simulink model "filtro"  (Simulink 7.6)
settings: Solver=ode45  StartTime=0.0  StopTime=100  MaxStep=0.1  RelTol=1e-3  AbsTol=1e-3

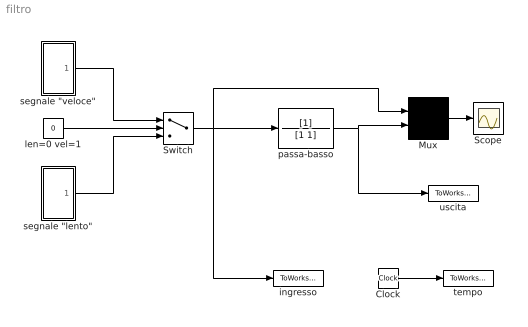
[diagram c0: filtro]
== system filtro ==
  Clock : Clock
  Mux : Mux  Inputs=2
  Scope : Scope
  Switch : Switch  Threshold=1
  ingresso : ToWorkspace  VariableName=u  SaveFormat=Array
  len=0 vel=1 : Constant  Value=0
  passa-basso : TransferFcn  Denominator=[1 1]
  "segnale \"lento\"" : Subsystem
  "segnale \"veloce\"" : Subsystem
  tempo : ToWorkspace  VariableName=t  SaveFormat=Array
  uscita : ToWorkspace  VariableName=yf  SaveFormat=Array
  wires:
  Mux/1 -> Scope/1
  Clock/1 -> tempo/1
  passa-basso/1 -> Mux/2, uscita/1
  len=0 vel=1/1 -> Switch/2
  "segnale \"veloce\""/1(out_1) -> Switch/1
  "segnale \"lento\""/1(out_1) -> Switch/3
  Switch/1 -> passa-basso/1, Mux/1, ingresso/1

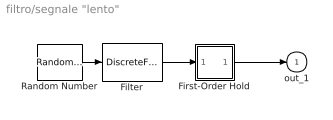
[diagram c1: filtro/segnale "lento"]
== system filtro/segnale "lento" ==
  Filter : DiscreteFilter  Denominator=[1 -0.9]  SampleTime=1
  First-Order Hold : Subsystem  mask(First-Order Hold){Ts=1}
      mask prompts: Ts "Sample Time:"
      mask help: First-Order Hold
  Random Number : RandomNumber  SampleTime=1
  out_1 : Outport
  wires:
  Random Number/1 -> Filter/1
  Filter/1 -> First-Order Hold/1(input)
  First-Order Hold/1(output) -> out_1/1

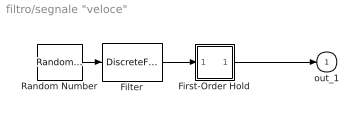
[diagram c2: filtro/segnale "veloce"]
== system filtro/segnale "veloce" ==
  Filter : DiscreteFilter  Denominator=[1 0.9]  SampleTime=1
  First-Order Hold : Subsystem  mask(First-Order Hold){Ts=1}
      mask prompts: Ts "Sample Time:"
      mask help: First-Order Hold
  Random Number : RandomNumber  SampleTime=1
  out_1 : Outport
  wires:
  Random Number/1 -> Filter/1
  Filter/1 -> First-Order Hold/1(input)
  First-Order Hold/1(output) -> out_1/1

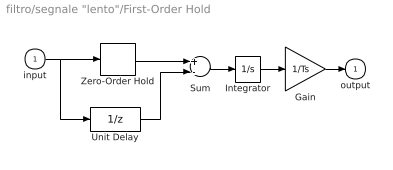
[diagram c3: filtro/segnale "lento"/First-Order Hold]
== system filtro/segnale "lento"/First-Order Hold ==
  input : Inport
  Gain : Gain  Gain=1/Ts
  Integrator : Integrator
  Sum : Sum  Inputs=+-
  Unit Delay : UnitDelay  SampleTime=Ts
  Zero-Order Hold : ZeroOrderHold  SampleTime=Ts
  output : Outport
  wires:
  input/1 -> Zero-Order Hold/1, Unit Delay/1
  Zero-Order Hold/1 -> Sum/1
  Unit Delay/1 -> Sum/2
  Sum/1 -> Integrator/1
  Integrator/1 -> Gain/1
  Gain/1 -> output/1

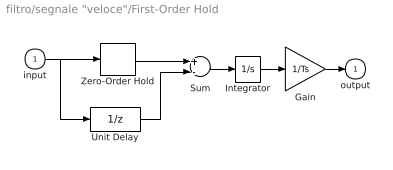
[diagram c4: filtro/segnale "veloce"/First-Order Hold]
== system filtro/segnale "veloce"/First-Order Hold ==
  input : Inport
  Gain : Gain  Gain=1/Ts
  Integrator : Integrator
  Sum : Sum  Inputs=+-
  Unit Delay : UnitDelay  SampleTime=Ts
  Zero-Order Hold : ZeroOrderHold  SampleTime=Ts
  output : Outport
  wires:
  input/1 -> Zero-Order Hold/1, Unit Delay/1
  Zero-Order Hold/1 -> Sum/1
  Unit Delay/1 -> Sum/2
  Sum/1 -> Integrator/1
  Integrator/1 -> Gain/1
  Gain/1 -> output/1
